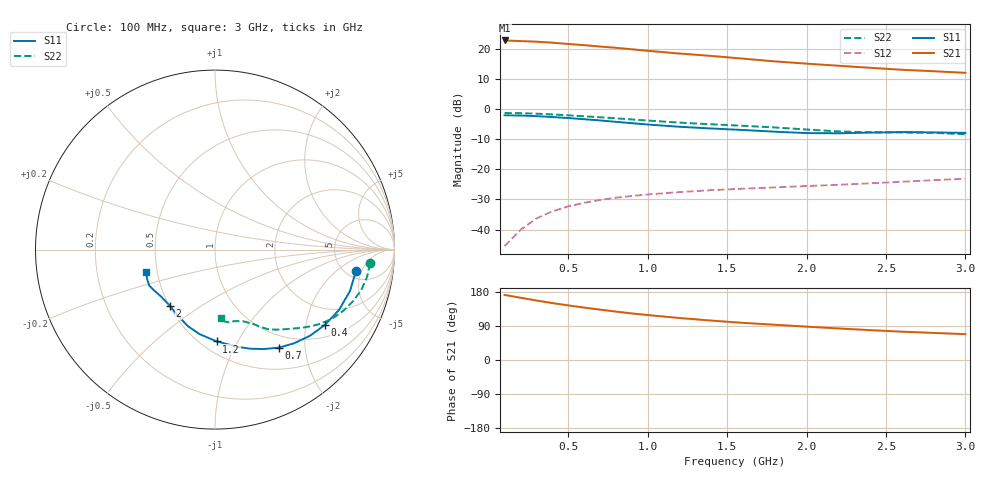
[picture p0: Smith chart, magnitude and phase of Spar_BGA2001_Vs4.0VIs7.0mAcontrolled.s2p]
! Filename: 47G1.001
! Title: BGA2001 X0297-20 HFE=80
! Bias: Vce=4V; Ic=7.0mA controlled / noise data included
! Company: NXP Semiconductors NL
! User: Quality&Reliability T&D
! Measure time: 23 Oct 1998 / 08:34:25
#  MHz  S  MA  R 50
! Freq  S11  S21  S12  S22  :
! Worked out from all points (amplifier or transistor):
!   20 points, 100 MHz to 3 GHz, reference 50 ohm
!   highest |S21| = 22.9 dB at 100 MHz (marker M1)
!   |S21| within 3 dB of that: start of sweep to 912.9 MHz
!   unconditionally stable (mu >= 1): 1.868 GHz to end of sweep
!   at 400 MHz: K = 0.34, MSG = 28.1 dB, |S12| = -34.0 dB
!   at 1.2 GHz: K = 0.68, MSG = 23.0 dB, |S12| = -27.6 dB
!   at 3 GHz: K = 1.25, MAG = 14.6 dB, |S12| = -23.1 dB
!   lowest NFmin = 1.45 dB at 1.8 GHz
!   S11 on the Smith chart (normalised r, x): 100 MHz: 6.16, -3.94; 400 MHz: 1.38, -2.58; 700 MHz: 0.81, -1.53; 1.2 GHz: 0.59, -0.82; 2 GHz: 0.50, -0.38; 3 GHz: 0.43, -0.13
100  0.7945 -8.5  13.94 171.7  0.005287 67.2  0.8669 -5.1
200  0.7866 -17.1  13.61 164.3  0.009872 74.9  0.8606 -10.3
300  0.7684 -25.9  13.29 157.1  0.01527 74.5  0.8447 -15.7
400  0.7426 -34.4  12.8 150.3  0.02003 71.4  0.8201 -20.7
500  0.7144 -42.2  12.19 144.1  0.02421 68.1  0.7937 -25.3
600  0.6833 -49.8  11.65 138.3  0.02787 65.2  0.7651 -29.3
700  0.6522 -56.8  11.05 133.0  0.03101 62.7  0.7364 -33.0
800  0.6179 -63.8  10.53 127.8  0.0338 60.5  0.7068 -36.2
900  0.5869 -70.2  9.942 122.9  0.03604 58.8  0.6776 -39.2
1000  0.558 -76.6  9.387 118.6  0.03827 57.5  0.6495 -42.1
1200  0.5116 -88.9  8.451 110.8  0.0419 55.5  0.5995 -47.6
1400  0.4791 -100.2  7.709 104.0  0.04516 54.4  0.5625 -52.5
1600  0.4521 -109.6  6.946 98.0  0.04777 54.5  0.5313 -56.5
1800  0.4239 -118.7  6.258 93.0  0.05023 55.6  0.4981 -59.7
2000  0.4018 -128.7  5.737 88.0  0.0528 55.9  0.4604 -63.4
2200  0.3983 -138.9  5.294 83.3  0.05553 56.1  0.4286 -68.7
2400  0.4093 -146.5  4.893 78.8  0.05862 57.0  0.413 -74.8
2600  0.4177 -151.4  4.539 74.8  0.06228 58.6  0.4115 -79.4
2800  0.4126 -156.1  4.29 71.5  0.06622 59.2  0.4052 -82.1
3000  0.4048 -162.0  4.036 68.2  0.06999 60.0  0.3845 -84.7
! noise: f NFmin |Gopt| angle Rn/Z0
900  1.47  0.26  20.2  0.3
1000  1.55  0.23  16.8  0.27
1800  1.45  0.239  72.9  0.263
2000  1.499  0.188  72.27  0.212
2200  1.612  0.167  82.61  0.213
2400  1.669  0.17  103.2  0.217
